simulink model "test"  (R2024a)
settings: Solver=FixedStepAuto  StartTime=0.0  StopTime=Inf  RelTol=1e-3  EnableMultiTasking=on
libraries: c2833xlib x1

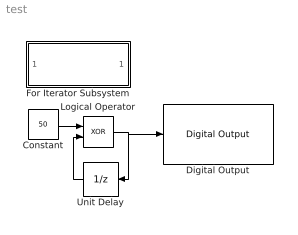
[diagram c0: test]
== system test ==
  Constant : Constant  Value=50
  Digital Output : c2833xlib/Digital Output  GPIO_Number=GPIO72~GPIO79  GPIO_Bit0=off  GPIO_BIT0_Toggle=off  GPIO_Bit1=off  GPIO_BIT1_Toggle=off  GPIO_Bit2=off  GPIO_BIT2_Toggle=off  GPIO_Bit3=on  GPIO_BIT3_Toggle=off  GPIO_Bit4=off  GPIO_BIT4_Toggle=off  GPIO_Bit5=off  GPIO_BIT5_Toggle=off  GPIO_Bit6=off  GPIO_BIT6_Toggle=off  GPIO_Bit7=off  GPIO_BIT7_Toggle=off
  For Iterator Subsystem : Subsystem  TreatAsAtomicUnit=on
  Logical Operator : Logic  Operator=XOR  AllPortsSameDT=off  OutDataTypeStr=boolean
  Unit Delay : UnitDelay  SampleTime=-1  HasFrameUpgradeWarning=on
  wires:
  Constant/1 -> Logical Operator/1
  Logical Operator/1 -> Digital Output/1, Unit Delay/1
  Unit Delay/1 -> Logical Operator/2

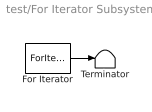
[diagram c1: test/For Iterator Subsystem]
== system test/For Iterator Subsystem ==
  For Iterator : ForIterator  IterationLimit=3000000
  Terminator : Terminator
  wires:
  For Iterator/1 -> Terminator/1
